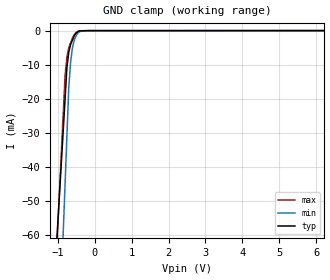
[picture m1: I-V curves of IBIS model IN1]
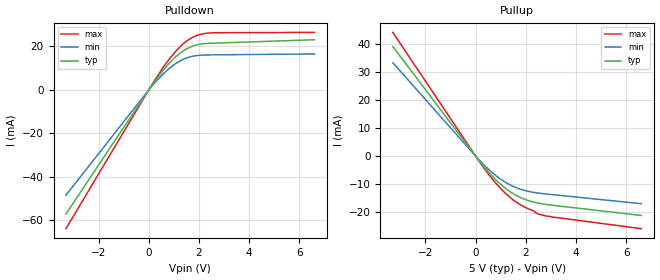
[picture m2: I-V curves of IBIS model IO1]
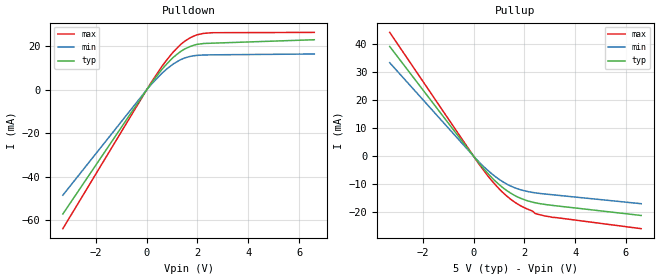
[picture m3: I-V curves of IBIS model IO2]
[IBIS Ver]   5.0
[File Name]   1273na065.ibs
[File Rev]   1.0
[Date]   October 11, 2019
[Source]   JSC NIIET
[Disclaimer]
|   IBIS MODEL LICENSE AND DISCLAIMER AGREEMENT
|  Before downloading or using the below-referenced IBIS model, please read and
|  accept the license agreement and disclaimer shown below.
|   LICENSE STATEMENT
|  The information in this IBIS model is protected under the copyright laws of
|  the Russia and other countries. JSC NIIET hereby
|  grants the users of this IBIS model (hereto referred to as licensee) a
|  nonexclusive, nontransferable license to use this IBIS model as long as the
|  licensee abides by the terms of this agreement.
|  Before using the IBIS model, the licensee should read this license. By using,
|  copying, modifying or redistributing this IBIS model,licensee accepts and
|  agrees to become bound by the terms of this agreement. If the licensee does
|  not accept these terms, then the licensee should not use the IBIS model and
|  should return it to JSC NIIET immediately.
|  The licensee may not sell, loan, rent, lease, distribute or license the IBIS
|  model,in whole, in part, or in modified form, to anyone outside the
|  licensee's company. The licensee may modify the IBIS model to suit his
|  specific applications, provided that all rights in such modifications and
|  derivative works shall belong to JSC NIIET. The licensee may make copies of this
|  IBIS model for use within his company only.
|  THIS IBIS MODEL IS PROVIDED AS IS, WHERE IS, AND WITH NO WARRANTY OF ANY
|  KIND EITHER EXPRESSED OR IMPLIED, INCLUDING BUT NOT LIMITED TO ANY IMPLIED
|  WARRANTIES OF MERCHANTABILITY AND FITNESS FOR A PARTICULAR PURPOSE.
|  Licensee understands that the mathematical behavioral characteristics and
|  formulas for the IBIS model have not been fully characterized for production
|  specification or exact compliance to actual part operation. The IBIS model
|  is useful for general simulations but not intended for safety critical,
|  manufacturing yield, or similar safety or financial decision making
|  simulations. In no event will JSC NIIET be liable for indirect, special,
|  collateral, incidental, consequential or punitive damages in connection with
|  or arising out of the use of this IBIS model. JSC NIIET reserves the right to
|  make changes to its products and the IBIS model without prior notice.
|  The Parties agree that the foregoing terms constitute the entire agreement
|  and that this agreement shall be governed by and construed in accordance
|  with the laws of the Russsia, without regard to choice of law provisions.
[Copyright]
|  This model is an exclusive property of JSC NIIET
|  and is not to be resold or redistributed without the written
|  permission of JSC NIIET.
|  Copyright(c) 2019 JSC NIIET, All Rights Reserved
|   Component 1273HA065
[Component]   1273HA065
[Manufacturer] JSC NIIET
[Package]
| variable   typ   min   max
R_pkg   0   NA   NA
L_pkg   0   NA   NA
C_pkg   0   NA   NA
[Pin]   signal_name   model_name   R_pin   L_pin   C_pin
1   AUXDATA1   TERM   NA   NA   NA
2   NC   NC   NA   NA   NA
3   AUXTDMBCLK   IO1   NA   NA   NA
4   AUXTDMLRCLK   IO1   NA   NA   NA
5   CIN   IN1   NA   NA   NA
6   COUT   IO2   NA   NA   NA
7   DGND   GND   NA   NA   NA
8   CCLK   IN1   NA   NA   NA
9   CLATCH#   IN1   NA   NA   NA
10   OL1   TERM   NA   NA   NA
11   OR1   TERM   NA   NA   NA
12   OL2   TERM   NA   NA   NA
13   OR2   TERM   NA   NA   NA
14   AGND   GND   NA   NA   NA
15   AVCC   POWER   NA   NA   NA
16   AGND   GND   NA   NA   NA
17   FILTR   TERM   NA   NA   NA
18   AGND   GND   NA   NA   NA
19   AVCC   POWER   NA   NA   NA
20   CM   TERM   NA   NA   NA
21   NC   NC   NA   NA   NA
22   NC   NC   NA   NA   NA
23   NC   NC   NA   NA   NA
24   NC   NC   NA   NA   NA
25   NC   NC   NA   NA   NA
26   NC   NC   NA   NA   NA
27   NC   NC   NA   NA   NA
28   NC   NC   NA   NA   NA
29   LF   TERM   NA   NA   NA
30   AVCC   POWER   NA   NA   NA
31   AGND   GND   NA   NA   NA
32   MCLKI/XI   XI   NA   NA   NA
33   MCLKO/XO   XO   NA   NA   NA
34   AGND   GND   NA   NA   NA
35   AVCC   POWER   NA   NA   NA
36   OL3   TERM   NA   NA   NA
37   OR3   TERM   NA   NA   NA
38   OL4   TERM   NA   NA   NA
39   OR4   TERM   NA   NA   NA
40   PD#/RST#   IN1   NA   NA   NA
41   DSDATA4   IO1   NA   NA   NA
42   DGND   GND   NA   NA   NA
43   DVCC   POWER   NA   NA   NA
44   DSDATA3   IO1   NA   NA   NA
45   DSDATA2   IO1   NA   NA   NA
46   DSDATA1   IO1   NA   NA   NA
47   DBCLK   IO1   NA   NA   NA
48   DLRCLK   IO1   NA   NA   NA
[Model]   TERM
Model_type Terminator
C_comp   0F   0F   0F
[Temperature Range]   25   -60   85
[Voltage Range]   5.00V   4.50V   5.50V
[POWER Clamp Reference]   5.00V   4.50V   5.50V
[GND Clamp Reference]   0.00V   0.00V   0.00V
| Models and submodels in the file (6): IN1 (Input), IO1 (I/O), IO2 (I/O), XI (Input), XO (Output), TERM (Terminator)
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[Model]   IN1
Model_type Input
Polarity   Non-Inverting
Vinl =   0.8V
Vinh =   2.1V
C_comp   7.970E-13F   7.970E-13F   7.970E-13F
[Temperature Range]   25   -60   85
[Voltage Range]   5.00V   4.50V   5.50V
[POWER Clamp Reference]   5.00V   4.50V   5.50V
[GND Clamp Reference]   0.00V   0.00V   0.00V
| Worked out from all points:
|   GND clamp passes 1 mA (typ) near -0.52 V on its own axis
[Power Clamp]
| Voltage   I(typ)   I(min)   I(max)
-3.3V     0A         0A         0A
0V        0A         0A         0A
6.6V      0A         0A         0A
[GND Clamp]
| Voltage   I(typ)   I(min)   I(max)
-3.3V     -484.3mA   -755.1mA   -576.1mA
-800mV    -20.08mA   -45.14mA   -13.05mA
-750mV    -10.79mA   -30.94mA   -7.71mA
-700mV    -6.308mA   -16.74mA   -4.984mA
-650mV    -4.076mA   -9.339mA   -3.551mA
-600mV    -2.756mA   -4.988mA   -2.118mA
-550mV    -1.435mA   -2.732mA   -1.158mA
-500mV    -712uA     -1.452mA   -512.7uA
-450mV    -271.7uA   -690.8uA   -161.3uA
-350mV    -54.63uA   -85.42uA   -25.58uA
-175mV    -889.4nA   -2.131uA   -2.047uA
6.6V      10.72uA    21.26uA    6.111uA
[Model]   IO1
Model_type I/O
Polarity   Non-Inverting
Vinl =   0.8V
Vinh =   2.1V
Vmeas =   1.65V
C_comp   7.970E-13F   7.970E-13F   7.970E-13F
[Temperature Range]   25   -60   85
[Voltage Range]   5.00V   4.50V   5.50V
[Pullup Reference]   5.00V   4.50V   5.50V
[Pulldown Reference]   0.00V   0.00V   0.00V
[POWER Clamp Reference]   5.00V   4.50V   5.50V
[GND Clamp Reference]   0.00V   0.00V   0.00V
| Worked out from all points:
|   slope of the pulldown table from 0 to 0.75 V, typ, clamps not added: 66 ohm
|   slope of the pullup table from 0 to 0.75 V, typ, clamps not added: 94.1 ohm
[Pullup]
| Voltage   I(typ)   I(min)   I(max)
-3.3V     39.14mA    33.34mA    44.17mA
240mV     -2.782mA   -2.293mA   -3.16mA
820mV     -8.605mA   -7.051mA   -9.819mA
1.12V     -11.01mA   -8.963mA   -12.72mA
1.46V     -13.21mA   -10.67mA   -15.39mA
1.9V      -15.22mA   -12.14mA   -17.97mA
2.32V     -16.43mA   -12.96mA   -19.64mA
2.42V     -16.64mA   -13.1mA    -20.45mA
2.8V      -17.24mA   -13.52mA   -21.39mA
6.6V      -21.19mA   -16.99mA   -25.9mA
[Pulldown]
| Voltage   I(typ)   I(min)   I(max)
-3.3V     -57.16mA   -48.5mA    -63.91mA
160mV     2.682mA    2.211mA    3.049mA
580mV     9.105mA    7.381mA    10.45mA
820mV     12.28mA    9.862mA    14.19mA
1.06V     15.07mA    11.99mA    17.56mA
1.4V      18.12mA    14.2mA     21.47mA
1.68V     19.79mA    15.29mA    23.74mA
1.88V     20.63mA    15.72mA    24.87mA
2.26V     21.33mA    16.03mA    26mA
6.6V      23.05mA    16.5mA     26.43mA
[Ramp]
| variable   typ   min   max
dV/dt_r   5.0125E-01/5.0539E-10   NA   NA
dV/dt_f   6.3759E-01/4.9067E-10   NA   NA
R_load = 50ohms
[Model]   IO2
Model_type I/O
Polarity   Non-Inverting
Vinl =   0.8V
Vinh =   2.1V
Vmeas =   1.65V
C_comp   7.970E-13F   7.970E-13F   7.970E-13F
[Temperature Range]   25   -60   85
[Voltage Range]   5.00V   4.50V   5.50V
[Pullup Reference]   5.00V   4.50V   5.50V
[Pulldown Reference]   0.00V   0.00V   0.00V
[POWER Clamp Reference]   5.00V   4.50V   5.50V
[GND Clamp Reference]   0.00V   0.00V   0.00V
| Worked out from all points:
|   slope of the pulldown table from 0 to 0.75 V, typ, clamps not added: 66 ohm
|   slope of the pullup table from 0 to 0.75 V, typ, clamps not added: 94.1 ohm
[Pullup]
| Voltage   I(typ)   I(min)   I(max)
-3.3V     39.14mA    33.34mA    44.17mA
240mV     -2.782mA   -2.293mA   -3.16mA
820mV     -8.605mA   -7.051mA   -9.819mA
1.12V     -11.01mA   -8.963mA   -12.72mA
1.46V     -13.21mA   -10.67mA   -15.39mA
1.9V      -15.22mA   -12.14mA   -17.97mA
2.32V     -16.43mA   -12.96mA   -19.64mA
2.42V     -16.64mA   -13.1mA    -20.45mA
2.8V      -17.24mA   -13.52mA   -21.39mA
6.6V      -21.19mA   -16.99mA   -25.9mA
[Pulldown]
| Voltage   I(typ)   I(min)   I(max)
-3.3V     -57.16mA   -48.5mA    -63.91mA
160mV     2.682mA    2.211mA    3.049mA
580mV     9.105mA    7.381mA    10.45mA
820mV     12.28mA    9.862mA    14.19mA
1.06V     15.07mA    11.99mA    17.56mA
1.4V      18.12mA    14.2mA     21.47mA
1.68V     19.79mA    15.29mA    23.74mA
1.88V     20.63mA    15.72mA    24.87mA
2.26V     21.33mA    16.03mA    26mA
6.6V      23.05mA    16.5mA     26.43mA
[Ramp]
| variable   typ   min   max
dV/dt_r   5.0E-01/5.0E-10   3.8E-01/5.0E-10   6.2E-01/4.7E-10
dV/dt_f   6.9E-01/4.9E-10   4.8E-01/5.2E-10   7.8E-01/4.6E-10
R_load = 50ohms
